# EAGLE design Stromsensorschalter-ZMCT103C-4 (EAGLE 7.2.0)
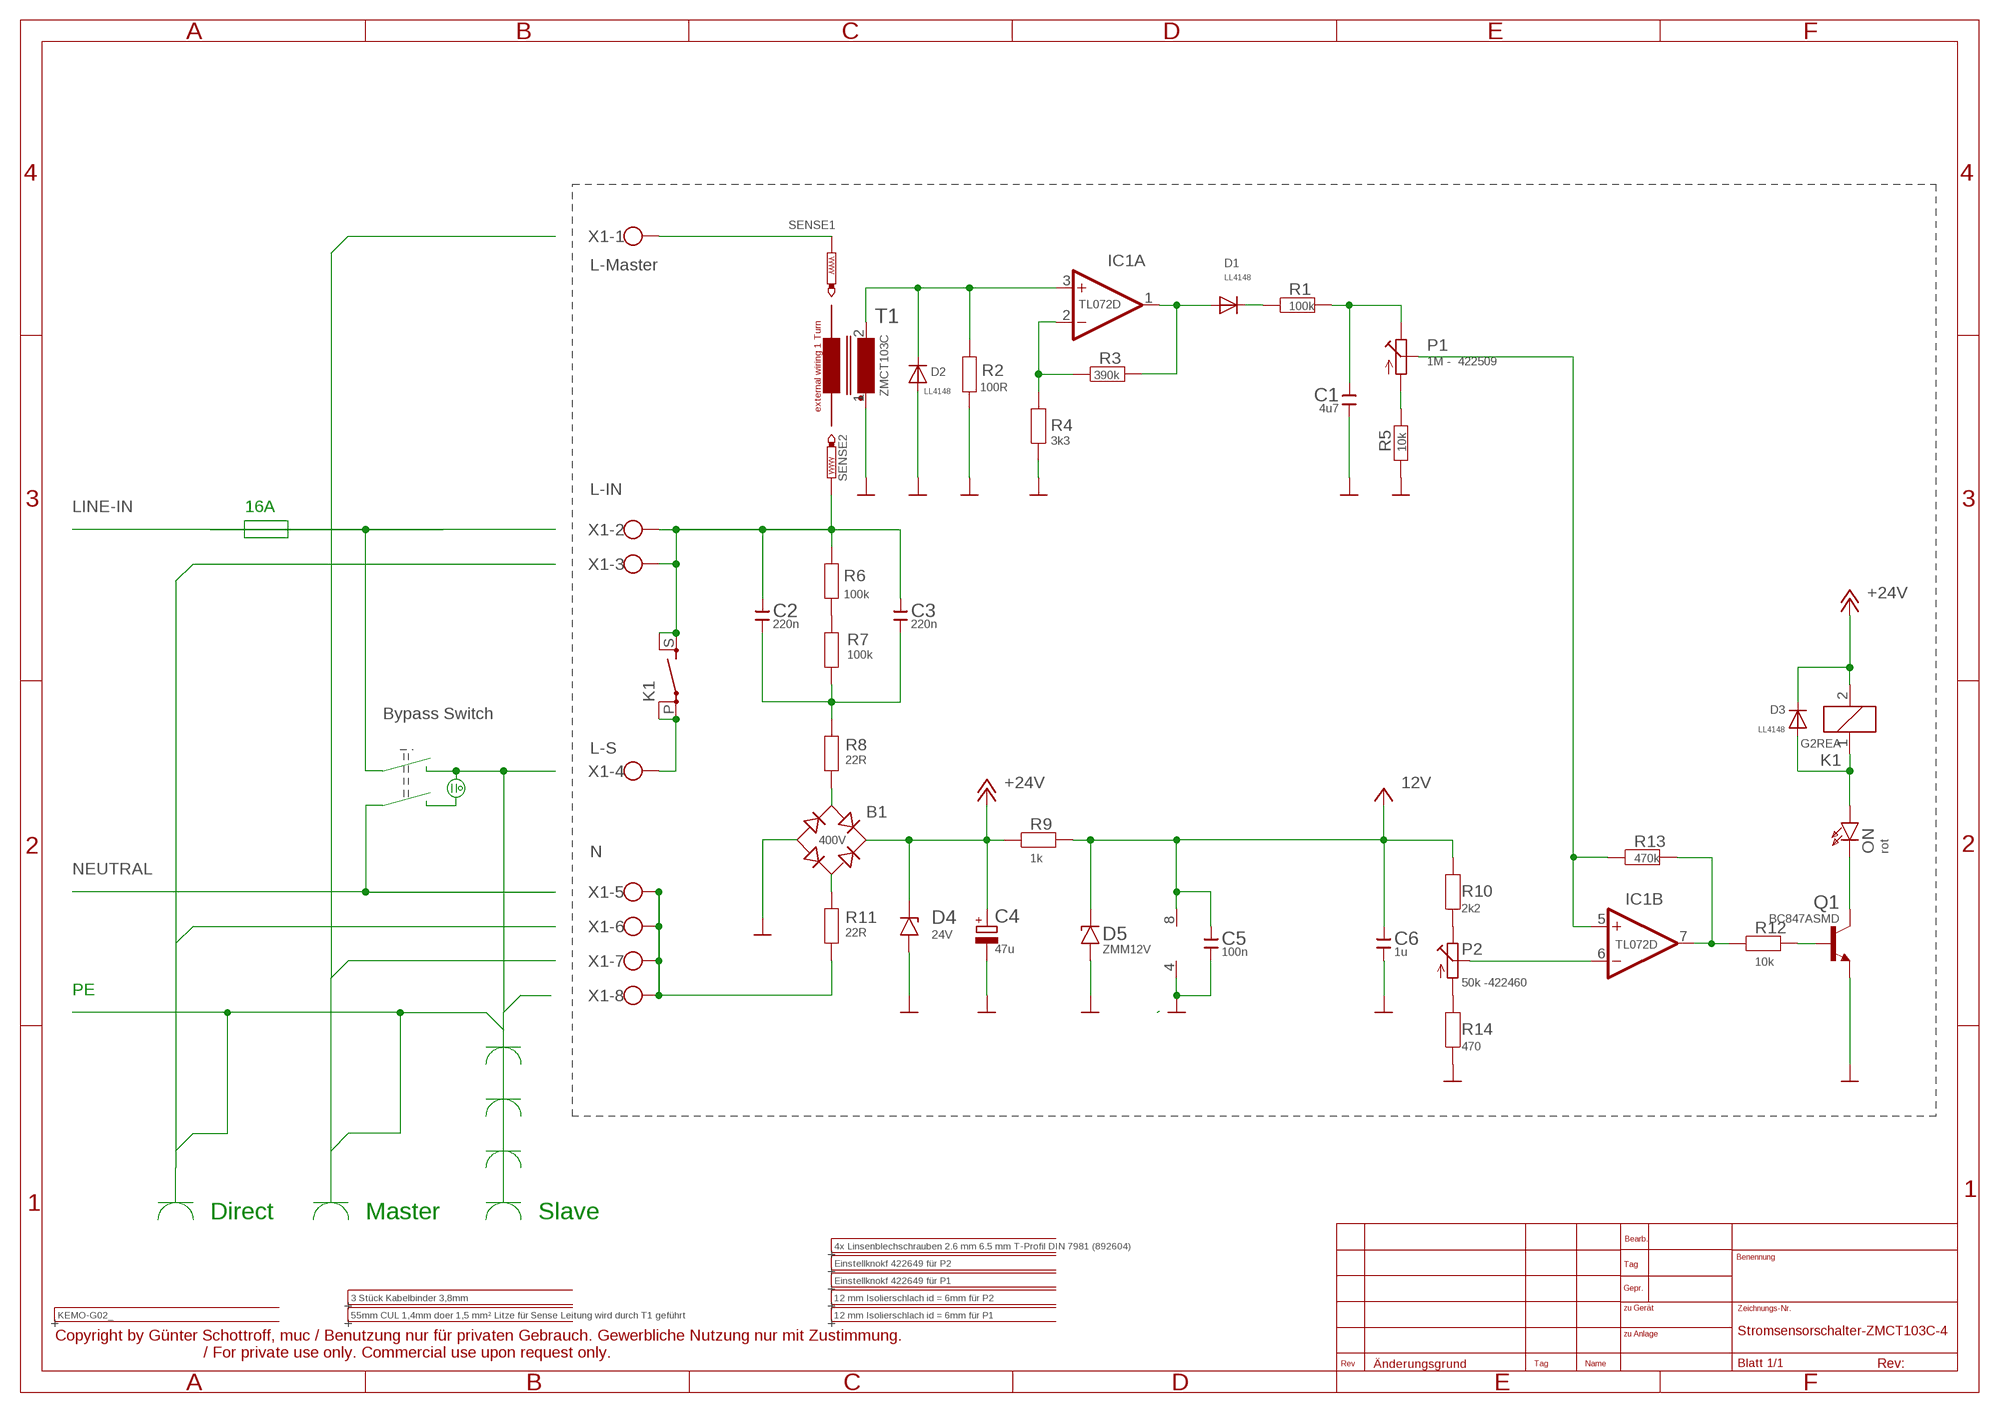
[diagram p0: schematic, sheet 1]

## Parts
..1  4x Linsenblechschrauben 2.6 mm 6.5 mm T-Profil DIN 7981 (892604)  INFO  [INFO]
..2  Einstellknokf 422649 für P2  INFO  [INFO]
..3  Einstellknokf 422649 für P1  INFO  [INFO]
..4  3 Stück Kabelbinder 3,8mm  INFO  [INFO]
..5  12 mm Isolierschlach id = 6mm für P2  INFO  [INFO]
..6  55mm CUL 1,4mm doer 1,5 mm² Litze für Sense Leitung wird durch T1 geführt  INFO  [INFO]
..7  12 mm Isolierschlach id = 6mm für P1  INFO  [INFO]
B1  400V  B-DILB-DIL_SMD  [B-DIL_SMD]
C1  4u7  C-EUC1210  [C1210]
C2  220n  C-EU150-072X183  [C150-072X183]
C3  220n  C-EU150-072X183  [C150-072X183]
C4  47u  CPOL-EUE5-8.5  [E5-8,5]
C5  100n  C-EUC1206  [C1206]
C6  1u  C-EUC1206  [C1206]
D1  LL4148  [1206]
D2  LL4148  [1206]
D3  LL4148  [1206]
D4  24V  ZENER-DIODEDO34-7  [DO34Z7]
D5  ZMM12V  ZENER-DIODESOD80C  [SOD80C]
ENCLOSURE-  KEMO-G02_  [KEMO-G02_]
IC1  TL072D  [SO08]
K1  G2REA  [G2REA]
ON  rot  LED5MM  [LED5MM]
P1  1M - 422509  TRIM_EU-CA6V  [CA6V]
P2  50k -422460  TRIM_EU-CA6V  [CA6V]
Q1  BC847ASMD  [SOT23]
R1  100k  R-EU_R1206  [1206]
R2  100R  R-EU_R1206  [1206]
R3  390k  R-EU_R1206  [1206]
R4  3k3  R-EU_R1206  [1206]
R5  10k  R-EU_R1206  [1206]
R6  100k  R-EU_R1206  [1206]
R7  100k  R-EU_R1206  [1206]
R8  22R  R-EU_R1206  [1206]
R9  1k  R-EU_R1206  [1206]
R10  2k2  R-EU_R1206  [1206]
R11  22R  R-EU_R1206  [1206]
R12  10k  R-EU_R1206  [1206]
R13  470k  R-EU_R1206  [1206]
R14  470  R-EU_R1206  [1206]
SENSE1  P1-13P-17  [P1-17]
SENSE2  P1-13P-17  [P1-17]
T1  ZMCT103C  [ZMCT103C]
X1  AK500/8  [AK500/8]

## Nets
12V: C5.1 C6.1 D5.C IC1.8(P:V+) R9.2 R10.2
+24V: B1.+ C4.+ D3.1 D4.C K1.2 R9.1
GND: B1.- C1.2 C4.- C5.2 C6.2 D2.2 D4.A D5.A IC1.4(P:V-) Q1.2(E) R2.2 R4.1 R5.1 R14.1 T1.1
L-IN: C2.1 C3.1 K1.S(2:S) K1.S@(2:S) R6.2 SENSE2.1(PS) X1.2 X1.3
L-S: K1.P(2:P) K1.P@(2:P) X1.4
N: R11.1 X1.5 X1.6 X1.7 X1.8
N$1: D2.1 IC1.3(A:+IN) R2.1 T1.2
N$2: ON.K(C) Q1.3(C)
N$3: D1.2 IC1.1(A:OUT) R3.2
N$4: IC1.2(A:-IN) R3.1 R4.2
N$5: C1.1 P1.E R1.2
N$6: IC1.7(B:OUT) R12.1 R13.2
N$7: SENSE1.1(PS) X1.1
N$8: IC1.6(B:-IN) P2.S
N$9: C2.2 C3.2 R7.1 R8.2
N$10: IC1.5(B:+IN) P1.S R13.1
N$11: B1.AC1 R11.2
N$12: Q1.1(B) R12.2
N$13: D3.2 K1.1 ON.A
N$14: R6.1 R7.2
N$15: B1.AC2 R8.1
N$16: P1.A R5.2
N$18: P2.E R10.1
N$19: P2.A R14.2
N$20: D1.1 R1.1

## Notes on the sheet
- L-Master
- 16A
- Bypass Switch
- PE
- Direct | Master | Slave

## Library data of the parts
..1-..7 = frames:INFO
B1 = rectifier:B-DIL: RECTIFIER
C1-C3 C5 C6 = rcl:C-EU: CAPACITOR, European symbol
C4 = rcl:CPOL-EU: POLARIZED CAPACITOR, European symbol
D1-D3 = allgem:LL4148
D4 D5 = diode:ZENER-DIODE: Z-Diode
ENCLOSURE- = Enclosures-DIN-Rail+more:KEMO-G02_; ENCLOSURES: ENCLOSURE-KEMO-G020,G024,G025,G026,G028
IC1 = linear:TL072: OP AMP
K1 = relay:G2REA: RELAY 1 x norm. open, high current, Omron
ON = led:LED: LED
P1 P2 = pot:TRIM_EU-: POTENTIOMETER
Q1 = transistor-npn:BC847*: NPN Transistor
R1-R14 = rcl:R-EU_: RESISTOR, European symbol
SENSE1 SENSE2 = testpad:P1-13: TEST PIN
T1 = INDUCT~3:ZMCT103C
X1 = con-ptr500:AK500/8: CONNECTOR

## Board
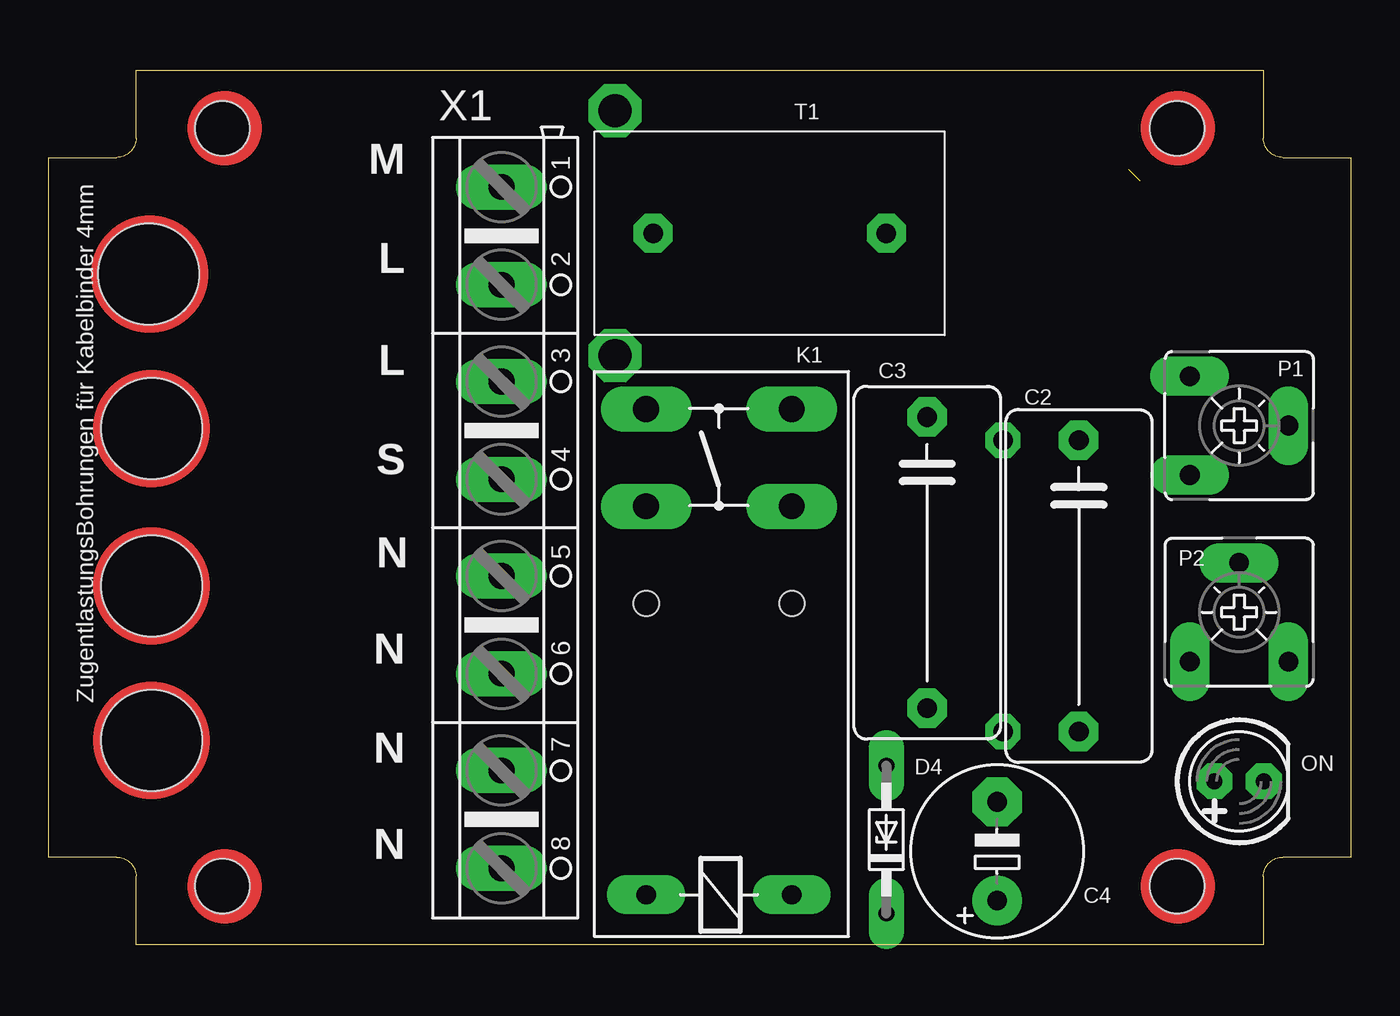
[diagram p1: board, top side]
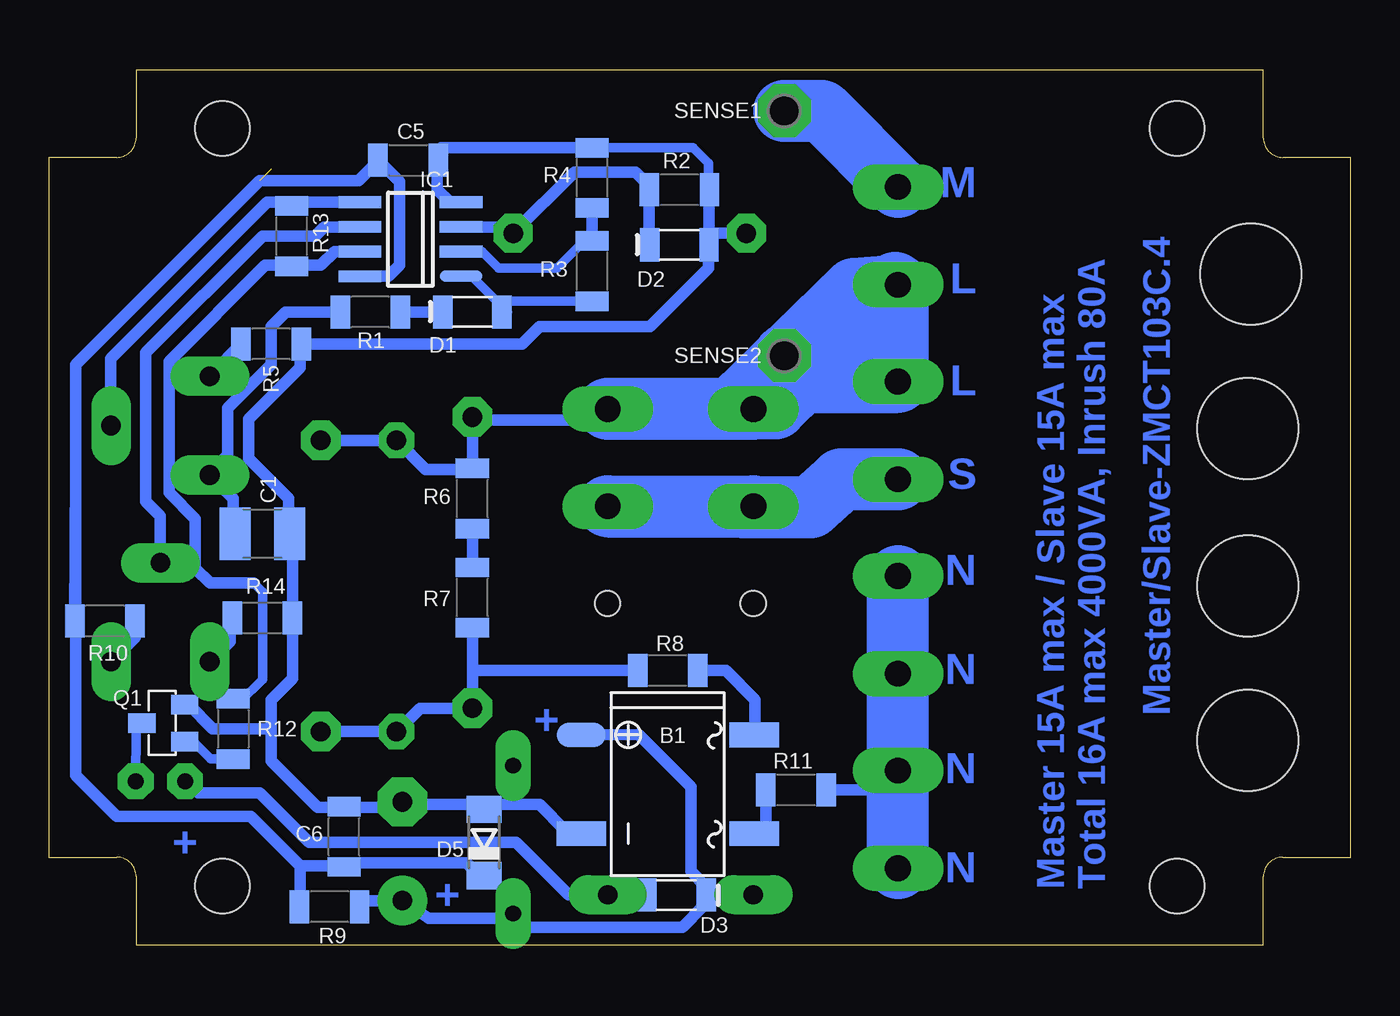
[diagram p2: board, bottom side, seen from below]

Size 67 x 45 mm. Coordinates in mm from the lower left corner, seen from the top.
Copper layers (1*16): Top 0.035mm / dielectric 1.5mm / Bottom 0.035mm
Design rules "default *": minimum track width 10mil, minimum drill 24mil, track to track 8mil, track to pad 8mil, pad to pad 8mil, via to via 8mil, smd to smd 8mil, copper to edge 40mil, drill to drill 8mil, minimum pad ring 20mil, minimum via ring 16mil, stop-mask expansion 0mil, vias tented up to drill 0mil, thermal gap 10mil
Holes 5.2 mm at 5.15,34.5 5.3,26.55 5.3,18.45 5.3,10.5

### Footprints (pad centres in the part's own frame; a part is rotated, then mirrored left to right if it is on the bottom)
B-DIL_SMD = smd 1.27 x 2.54: + -2.54,-4.445; - 2.54,-4.445; AC1 2.54,4.445; AC2 -2.54,4.445
C1210 = smd 1.6 x 2.7: 1 -1.4,0; 2 1.4,0
C150-072X183 = drill 1.016 octagon: 1 -7.493,0; 2 7.493,0
E5-8,5 = drill 1.016 pad 2.54: + -2.54,0 | drill 1.016 pad 2.54 octagon: - 2.54,0
C1206 = smd 1 x 1.7: 1 -1.55,0; 2 1.55,0
1206 = smd 1 x 1.7: 1 -1.525,0; 2 1.525,0
DO34Z7 = drill 0.813 long: A 3.81,0; C -3.81,0
SOD80C = smd 1.4 x 1.8: A 1.7,0; C -1.7,0
KEMO-G02_ = hole 2.8: -24.55,19.5; 24.55,19.5; 24.55,-19.5; -24.55,-19.5
SO08 = smd 0.6 x 2.2: 1 -1.905,-2.6; 2 -0.635,-2.6; 3 0.635,-2.6; 4 1.905,-2.6; 5 1.905,2.6; 6 0.635,2.6; 7 -0.635,2.6; 8 -1.905,2.6
G2REA = drill 1 long: 1 -2.54,-3.683; 2 -2.54,3.81 | drill 1.321 long: P 17.45,-3.683; P@ 17.45,3.81; S 22.454,-3.683; S@ 22.454,3.81 | hole 1.3: 12.45,3.8; 12.45,-3.7
LED5MM = drill 0.813 pad 1.676 octagon: A -1.27,0; K 1.27,0
CA6V = drill 1.016 long: A -2.54,-2.54; E 2.54,-2.54; S 0,2.54
SOT23 = smd 1 x 1.4: 1 -0.95,-1.1; 2 0.95,-1.1; 3 0,1.1
1206' = smd 1 x 1.7: 1 -1.55,0; 2 1.55,0
P1-17 = drill 1.702 pad 2.54 octagon: 1 0,0
ZMCT103C = drill 1 octagon: 1 -6,0; 2 6,0
AK500/8 = drill 1.321 long: 1 -17.526,0; 2 -12.497,0; 3 -7.518,0; 4 -2.489,0; 5 2.489,0; 6 7.518,0; 7 12.497,0; 8 17.526,0

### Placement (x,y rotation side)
..1  not placed on the board
..2  not placed on the board
..3  not placed on the board
..4  not placed on the board
..5  not placed on the board
..6  not placed on the board
..7  not placed on the board
B1  35.15,8.25 270 bottom
C1  56,21.15 0 bottom
C2  53,18.45 270 top
C3  45.2,19.65 270 top
C4  48.8,4.8 90 top
C5  48.5,40.35 0 bottom
C6  51.8,5.55 90 bottom
D1  45.2,32.55 0 bottom
D2  34.55,36 0 bottom
D3  34.7,2.55 180 bottom
D4  43.1,5.4 90 top
D5  44.6,5.25 90 bottom
ENCLOSURE-  33.5,22.5 0 top
IC1  48.38,36.29 90 bottom
K1  34.55,5.1 90 top
ON  61.25,8.4 0 top
P1  61.25,26.7 270 top
P2  61.25,17.1 0 top
Q1  61.1,11.4 90 bottom
R1  100k  [1206']  50.45,32.55 180 bottom
R2  100R  [1206']  34.55,38.85 0 bottom
R3  390k  [1206']  39.05,34.65 270 bottom
R4  3k3  [1206']  39.05,39.45 270 bottom
R5  10k  [1206']  55.55,30.9 180 bottom
R6  100k  [1206']  45.2,22.95 90 bottom
R7  100k  [1206']  45.2,17.85 90 bottom
R8  22R  [1206']  35.15,14.1 180 bottom
R9  1k  [1206']  52.55,1.95 180 bottom
R10  2k2  [1206']  64.1,16.65 180 bottom
R11  22R  [1206']  28.55,7.95 180 bottom
R12  10k  [1206']  57.5,11.1 270 bottom
R13  470k  [1206']  54.5,36.45 270 bottom
R14  470  [1206']  56,16.8 180 bottom
SENSE1  29.15,42.9 0 bottom
SENSE2  29.15,30.3 0 bottom
T1  37.1,36.6 0 top
X1  23.3,21.45 270 top

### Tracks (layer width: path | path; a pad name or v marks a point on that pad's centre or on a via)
12V  (1 unrouted)
  Bottom 0.6: 65.6,24.45 65.6,29.85 56.15,39.3 51.05,39.3 50.05,40.3 C5.1 48.95,39.25 48.95,34.95 49.52,34.38 IC1.8 | 65.6,24.45 65.6,8.7 63.5,6.6 56.6,6.6 54.05,4.05 | R10.2 65.6,24.45 | D5.C 44.85,3.55 45.5,4.2 51.55,4.2 C6.1 51.85,4.05 54.05,4.05 | R9.2 54.1,2.05 54.05,2.25 54.05,4.05
+24V
  Bottom 0.6: D3.1 33.32,1.98 34.4,0.9 42.63,0.9 D4.C 43.31,1.59 43.55,1.35 47.44,1.35 C4.+ 50.99,2.26 R9.1 | B1.+ 36.66,10.81 33.95,8.1 33.95,3.77 33.2,3 33.17,2.98 D3.1 | D3.1 31.2,2.55 K1.2
GND
  Bottom 0.5: R4.1 33.85,41 33.05,40.2 33.05,38.9
  Bottom 0.6: T1.1 32.87,36.6 D2.2 | D2.2 33.02,38.67 R2.2 33.05,38.9 | D2.2 33.05,36.72 33.05,34.8 36.05,31.8 41.75,31.8 42.65,30.9 R5.1 54.05,30.85 54.05,29.7 56.7,27.05 56.7,25 54.65,22.95 54.65,21.2 C1.2 54.45,21 R14.1 54.45,13.7 55.55,12.6 55.55,11.1 | 55.55,11.1 55.55,9.45 53.15,7.05 51.7,7.05 C6.2 51.25,7.1 51.2,7.05 48.34,7.05 C4.- 48.19,7.2 45.2,7.2 44.9,7.05 D5.A 45,6.95 45.05,7.2 42.95,7.2 | 42.95,7.2 41.75,7.2 40.4,5.85 39.73,5.85 B1.- | D4.A 43.1,7.35 42.95,7.2 | Q1.2 59.8,12.35 58.55,11.1 55.55,11.1 | IC1.4 46.34,38.2 47,38.85 47,40.3 C5.2 47,40.4 47,40.8 46.8,41 R4.1
L-IN  (via drill 1)
  Bottom 0.6: SENSE2.1 31.19,28.26 K1.S@ 38.26,27.5 38.41,27.86 39.65,27 45.19,27 C3.1 R6.2 45.25,24.45 47.6,24.45 v49.1,25.95 v49.11,25.94 C2.1
  Bottom 3.2: K1.S@ K1.S | 31.25,27.6 29.6,27.6 | 28.25,28.95 29.6,27.6 | 29.6,27.6 29.3,29.7 31.1,27.9 31.7,27.75 25.55,33.75 23.6,33.9 23.45,34.05 SENSE2.1 29.6,27.6 | 23.3,33.9 28.25,28.95 | 28.25,28.95 23.3,28.95 X1.3 X1.2
L-S
  Bottom 3.2: X1.4 26.21,23.94 27.8,22.5 31.27,22.5 K1.P K1.P@
N
  Bottom 0.6: X1.7 24.3,7.95 R11.1
  Bottom 3.2: X1.8 X1.7 X1.6 X1.5
N$1
  Bottom 0.6: D2.1 36.1,36.48 R2.1 36.1,39.05 36.8,39.75 39.95,39.75 T1.2 43.72,36.92 IC1.3
N$2
  Bottom 0.5: Q1.3 62.5,11.07 ON.K
N$3
  Bottom 0.5: R3.2 43.32,33.1 D1.2 43.4,32.55 45.23,34.38 IC1.1
N$4
  Bottom 0.5: IC1.2 44.7,35.66 43.85,34.8 40.85,34.8 39.5,36.15
  Bottom 0.6: R4.2 R3.1 38.95,36.15 39.5,36.15
N$5
  Bottom 0.6: C1.1 57.5,21.25 57.5,22.95 P1.E 58.71,24.29 57.8,25.2 57.8,27.6 55.55,29.85 55.55,31.8 54.8,32.55 R1.2
N$6
  Bottom 0.5: R12.1 57.2,12.45 56,13.65 56,18.15 56.45,18.6
  Bottom 0.6: 56.45,18.6 58.7,18.6 59.45,19.35 59.45,21.9 60.8,23.25 60.8,30 55.85,34.95 54.55,34.95 R13.2 54.45,34.95 53,34.95 52.29,35.66 IC1.7
N$7
  Bottom 3.2: SENSE1.1 27.22,42.9 X1.1
N$8
  Bottom 0.6: P2.S 61.25,22.05 62,22.8 62,30.45 56,36.45 53.3,36.45 52.82,36.92 IC1.6
N$9  (via drill 1)
  Bottom 0.6: R7.1 45.2,14.1 | 45.2,14.1 C3.2 47.9,12.15 v49.1,10.95 v49.11,10.96 C2.2 | R8.2 45.2,14.1
N$10
  Bottom 0.6: IC1.5 54.5,38.2 | P1.S 63.8,30.15 55.75,38.2 54.5,38.2 | 54.5,38.2 R13.1
N$11
  Bottom 0.6: R11.2 30.1,5.87 B1.AC1
N$12
  Bottom 0.5: R12.2 58.65,9.55 59.45,10.35 Q1.1
N$13
  Bottom 0.6: D3.2 38.8,2.55 38.79,2.56 38.31,2.56 | ON.A 59.9,8.4 59.3,7.8 56.15,7.8 53.6,5.25 42.95,5.25 40.25,2.55 38.32,2.55 38.31,2.56 | K1.1 38.31,2.56
N$14
  Bottom 0.6: R7.2 R6.1
N$15
  Bottom 0.6: R8.1 32.15,14.1 30.65,12.6 30.65,10.85 B1.AC2
N$16
  Bottom 0.6: R5.2 58.6,29.35 P1.A
N$18
  Bottom 0.6: R10.1 62.55,15.8 P2.E
N$19
  Bottom 0.6: P2.A 58.69,14.56 57.65,15.6 57.65,16.5 R14.2
N$20
  Bottom 0.6: D1.1 R1.1
(copper drawn outside any net)
  shapes: Bottom circle x2, Top circle x8

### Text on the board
Bottom: M | Master/Slave-ZMCT103C.4 | L | L | S | N | N | + | N | N | + | Master 15A max / Slave 15A max / Total 16A max 4000VA, Inrush 80A | +
tPlace: M | ZugentlastungsBohrungen für Kabelbinder 4mm | L | L | S | N | N | N | N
